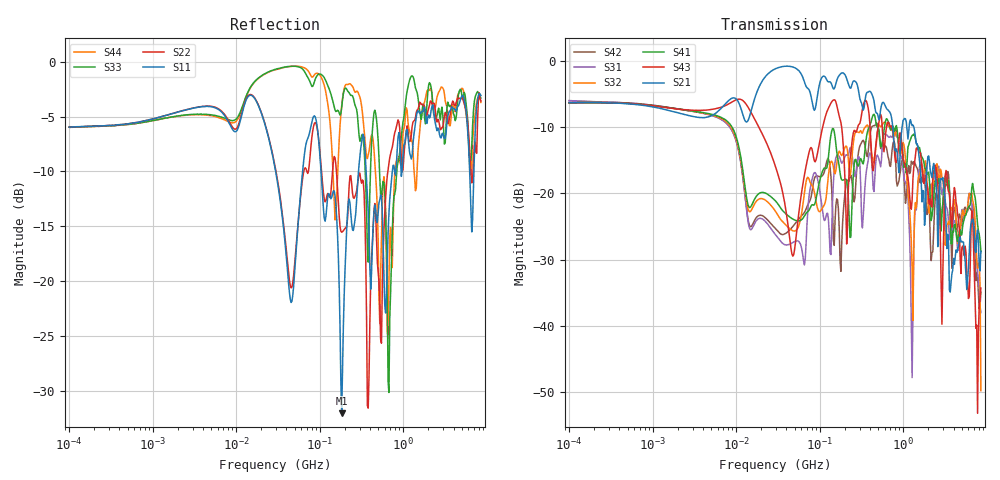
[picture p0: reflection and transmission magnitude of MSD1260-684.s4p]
# MHz S MA R 50
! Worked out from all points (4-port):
!   498 points, 100 kHz to 8.5 GHz, reference 50 ohm
!   strongest paths, dB at 100 kHz, 1.698 MHz, 29.49 MHz, 500.7 MHz, 8.5 GHz:
!     S21: -6.3, -7.6, -1.2, -8.4, -28.7
!     S43: -6.3, -7.2, -15.9, -10.0, -34.3
!     S41: -6.3, -7.1, -21.1, -10.1, -28.8
!     S32: -6.3, -7.1, -22.7, -10.0, -49.7
!     S31: -6.0, -7.1, -26.2, -14.4, -38.0
!     S42: -6.0, -7.1, -25.3, -10.0, -34.9
!   lowest |S11| = -32.1 dB at 183.3 MHz (marker M1), VSWR 1.05, Z = 48.3 + j1.74 ohm
!   |S11| at or under -10 dB: 103.7 MHz to 291.4 MHz (187.7 MHz wide, 95 % of centre); 359.3 MHz to 740.2 MHz (380.9 MHz wide, 69.3 % of centre); 6.236 GHz to 7.015 GHz (779.2 MHz wide, 11.8 % of centre)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
0.1  0.5033 7.4  0.4824 6.2  0.4999 -8.3  0.482 -174.8
     0.4824 6.2  0.5028 7.4  0.4818 -174.6  0.501 -8.3
     0.4999 -8.3  0.4818 -174.6  0.5029 7.4  0.4827 6.1
     0.482 -174.8  0.501 -8.3  0.4827 6.1  0.5026 7.5
86.26428  0.5669 -27.7  0.4235 -14.6  0.1435 77.6  0.08201 62.0
          0.4235 -14.6  0.5234 -8.7  0.1021 -75.3  0.1293 76.5
          0.1435 77.6  0.1021 -75.3  0.8096 -19.8  0.1758 25.5
          0.08201 62.0  0.1293 76.5  0.1758 25.5  0.8714 -30.5
183.289  0.02493 133.7  0.8101 -32.3  0.1693 35.1  0.1267 -6.7
         0.8101 -32.3  0.167 -36.6  0.1932 55.7  0.04137 66.1
         0.1693 35.1  0.1932 55.7  0.62 -32.5  0.3149 -60.7
         0.1267 -6.7  0.04137 66.1  0.3149 -60.7  0.6297 -5.9
673.7244  0.2022 -13.9  0.4172 -116.0  0.2652 -66.3  0.3386 -68.1
          0.4172 -116.0  0.3444 -12.8  0.3184 -77.3  0.1791 -84.4
          0.2652 -66.3  0.3184 -77.3  0.03102 -28.8  0.3391 -85.6
          0.3386 -68.1  0.1791 -84.4  0.3391 -85.6  0.09862 -38.0
1277.015  0.3738 -110.8  0.3245 -172.0  0.004088 -167.4  0.2739 -133.2
          0.3245 -172.0  0.5064 -111.5  0.02747 160.2  0.1725 -140.6
          0.004088 -167.4  0.02747 160.2  0.8631 -123.4  0.0888 -108.0
          0.2739 -133.2  0.1725 -140.6  0.0888 -108.0  0.4388 -140.5
2110.57  0.5651 -164.9  0.1465 106.5  0.109 165.9  0.08792 99.7
         0.1465 106.5  0.6624 -171.3  0.08174 168.6  0.04284 96.5
         0.109 165.9  0.08174 168.6  0.7908 -178.9  0.0906 134.5
         0.08792 99.7  0.04284 96.5  0.0906 134.5  0.7535 -169.0
8500  0.7015 -51.6  0.03679 -83.7  0.01264 -109.1  0.0364 -133.9
      0.03679 -83.7  0.6631 -42.6  0.003259 -120.4  0.01803 -92.1
      0.01264 -109.1  0.003259 -120.4  0.6826 -53.5  0.01934 -4.0
      0.0364 -133.9  0.01803 -92.1  0.01934 -4.0  0.6523 -55.6
